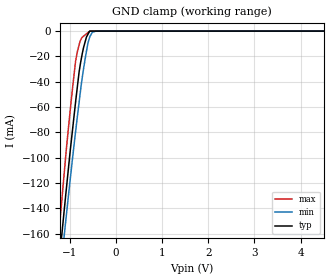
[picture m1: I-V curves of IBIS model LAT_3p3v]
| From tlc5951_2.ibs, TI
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|NOTES   Model TERM split into two Models TERM_3p3
|   and TERM_5p0 to accomodate vast voltage range of 3.0V - 5.5V
|   TERM_3p3 operates in voltage range of 3.0 - 3.3 - 3.6
|   TERM_5p0 operates in voltage range of 4.5 - 5.0 - 5.5
|   lat_3p3v Model
[Model]   LAT_3p3v
Model_type   Input
Vinl = 0.99
Vinh = 2.31
|   typ   min   max
|   (nom PVT)   (Fast PVT)   (slow PVT)
|Average
C_comp   1.254e-12   1.252e-12   1.266e-12
| Where nom  PVT is Nominal Process,  3.3V,  65C
|   Fast PVT is Strong Process,   3.6V,  -40C
|   Slow PVT is Weak Process,   3V,  125C
[Model Spec]
Vinl   0.99   0.9   1.08
Vinh   2.31   2.1   2.52
[Voltage Range]   3.3   3   3.6
|Ambient Temperature   25   85   -40
|Junction Temperature
[Temperature Range]   65   125   -40
[Power Clamp Reference]   3.3   3   3.6
[GND Clamp Reference]   0   0   0
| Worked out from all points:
|   GND clamp passes 1 mA (typ) near -0.58 V on its own axis
[GND Clamp]
|   Voltage   I(typ)   I(min)   I(max)
-3.3V     -1.048A    -1.001A    -1.101A
-1.255V   -192.9mA   -209.8mA   -168.9mA
-1.215V   -177.5mA   -195.4mA   -152.1mA
-1.122V   -142.7mA   -162.6mA   -113.5mA
-1.082V   -128.2mA   -149mA     -97.37mA
-870mV    -55.26mA   -78.66mA   -23.33mA
-795.3mV  -32.04mA   -55.94mA   -10.72mA
-726mV    -17.47mA   -36.15mA   -4.782mA
-636.9mV  -4.695mA   -15.98mA   -2.147mA
-567mV    0A         -4.755mA   -201.4uA
-417mV    0A         0A         0A
6.6V      0A         0A         0A
[POWER Clamp]
|   Voltage   I(typ)   I(min)   I(max)
-3.3V     0A         0A         0A
6.6V      0A         0A         0A
